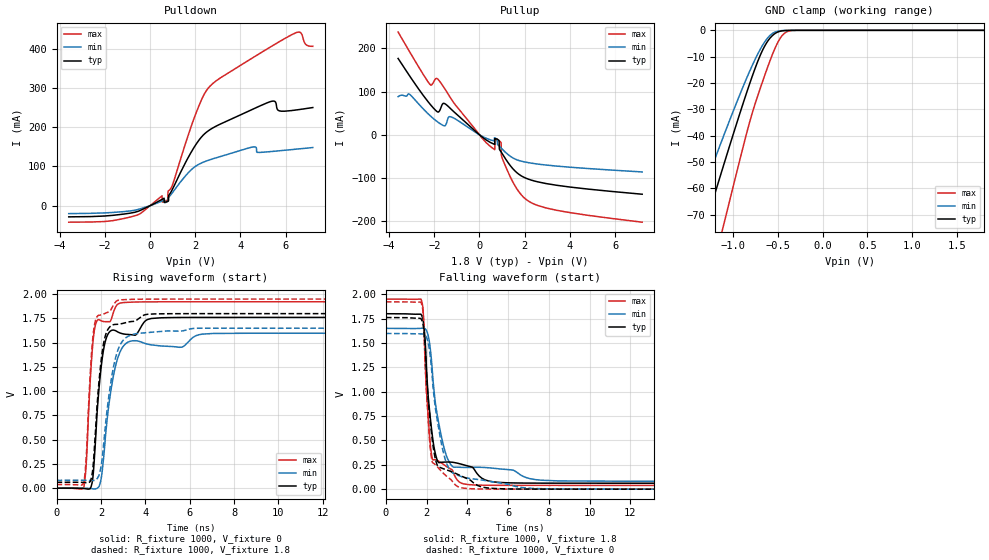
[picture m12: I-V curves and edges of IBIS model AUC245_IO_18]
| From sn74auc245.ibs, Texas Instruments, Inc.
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[Model]   AUC245_IO_18
Model_type  3-state
Enable   Active-Low
Vref =   0
Rref =   1000
Cref =   30p
Vmeas =   0.9
| variable   typ   min   max
C_comp   6.62pF   5.91pF   6.95pF
| C_pullup   7.05pF   0.21pF   13.03pF
| C_pulldown   7.18pF   2.24pF   14.68pF
| C_tri-state   6.62pF   5.91pF   6.95pF
[Temperature Range]   40   100   -40
| Ambient temperature   25   85   -40
[Voltage range]   1.8   1.65   1.95
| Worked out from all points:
|   slope of the pulldown table from 0 to 0.27 V, typ, clamps not added: 34.2 ohm
|   slope of the pullup table from 0 to 0.27 V, typ, clamps not added: 24.6 ohm
|   GND clamp passes 1 mA (typ) near -0.52 V on its own axis
|   rising waveform, R_fixture 1000, V_fixture 0: 20-80 % time 388ps typ, 555ps min, 285ps max; typ from 0 V to 1.76 V
|   falling waveform, R_fixture 1000, V_fixture 1.8: 20-80 % time 438ps typ, 661ps min, 314ps max; typ from 1.8 V to 0.061 V
|   rising waveform, R_fixture 1000, V_fixture 1.8: 20-80 % time 385ps typ, 555ps min, 280ps max; typ from 0.061 V to 1.8 V
|   falling waveform, R_fixture 1000, V_fixture 0: 20-80 % time 445ps typ, 672ps min, 313ps max; typ from 1.76 V to 0 V
[GND Clamp]
| AUC245_IO_18
|   Voltage   I(typ)   I(min)   I(max)
-3.6V     -336.3mA   -280.4mA   -411.7mA
-1.475V   -92.51mA   -73.75mA   -124.5mA
-1.34V    -77.23mA   -61.22mA   -106mA
-1.295V   -72.17mA   -57.08mA   -99.79mA
-1.1V     -50.45mA   -39.48mA   -72.99mA
-830mV    -21.69mA   -16.64mA   -36.59mA
-680mV    -8.152mA   -6.159mA   -20.29mA
-600mV    -3.457mA   -2.337mA   -12.58mA
-520mV    -951.5uA   -506.2uA   -5.863mA
-420mV    -86.5uA    -50.43uA   -943.1uA
-300mV    -2.47uA    -3.001uA   -18.45uA
1.8V      714.1pA    50.2nA     788.2pA
[Pulldown]
| AUC245_IO_18
|   Voltage   I(typ)   I(min)   I(max)
-3.6V     -28.49mA   -20.22mA   -42.08mA
-1.155V   -21.32mA   -15.05mA   -32.66mA
530mV     16.28mA    11.83mA    25.26mA
780mV     11.04mA    10.74mA    14.1mA
800mV     11.66mA    11.63mA    36.72mA
1.97V     150.9mA    98.78mA    226.4mA
2.645V    193.6mA    117.1mA    304.4mA
4.56V     246.4mA    149.8mA    377.8mA
5.38V     266.3mA    138.2mA    406.7mA
5.71V     242mA      140mA      417.9mA
6.445V    244mA      144mA      440.9mA
7.2V      250.3mA    148.3mA    406.4mA
[Pullup]
| AUC245_IO_18
|   Voltage   I(typ)   I(min)   I(max)
-3.6V     176.5mA    88.25mA    237.5mA
-2.185V   70.84mA    44.34mA    116.3mA
-1.835V   52.55mA    29.22mA    128.3mA
-1.53V    71.89mA    20.76mA    106.1mA
-1.26V    59.61mA    41.57mA    83.77mA
480mV     -17.54mA   -11.58mA   -26.82mA
845mV     -12.04mA   -24.63mA   -13.29mA
940mV     -38.16mA   -29.53mA   -16.81mA
980mV     -41.36mA   -31.67mA   -49.57mA
1.26V     -63.84mA   -45.45mA   -85.39mA
2.065V    -100.5mA   -63.4mA    -149.4mA
7.2V      -137.3mA   -85.82mA   -202mA
[Ramp]
| AUC245_IO_18
| variable   typ   min   max
dV/dt_r   1.06/3.92E-10   0.96/5.60E-10   1.16/2.93E-10
dV/dt_f   1.04/4.43E-10   0.94/6.67E-10   1.15/3.23E-10
R_load = 1000
[Rising Waveform]
| AUC245_IO_18
R_fixture =   1000
C_fixture =   0
L_fixture =   0
V_fixture =   0
V_fixture_min = 0
V_fixture_max = 0
|   Time   V(typ)   V(min)   V(max)
0s        11.26nV    38.5nV     1.726nV
1.235ns   -3.215mV   815.2uV    15.23mV
1.335ns   -6.28mV    825.8nV    235.8mV
1.625ns   82.37mV    -5.697mV   1.463V
1.92ns    1.041V     19.16mV    1.737V
2.26ns    1.559V     662.8mV    1.717V
2.55ns    1.63V      1.141V     1.803V
2.86ns    1.6V       1.404V     1.908V
7.04ns    1.761V     1.595V     1.922V
34.99ns   1.761V     1.597V     1.922V
[Falling Waveform]
| AUC245_IO_18
R_fixture =   1000
C_fixture =   0
L_fixture =   0
V_fixture =   1.8
V_fixture_min = 1.65
V_fixture_max = 1.95
|   Time   V(typ)   V(min)   V(max)
0s        1.8V       1.65V      1.95V
1.725ns   1.793V     1.65V      1.948V
1.83ns    1.729V     1.651V     1.824V
2.065ns   985.1mV    1.584V     785.7mV
2.28ns    548.4mV    1.211V     309.5mV
2.545ns   285.7mV    734mV      292mV
2.945ns   278.3mV    358.7mV    236.6mV
3.805ns   250.2mV    223mV      54.87mV
6ns       65.19mV    200.6mV    39.11mV
34.99ns   61.1mV     81.05mV    38.7mV
[Rising Waveform]
| AUC245_IO_18
R_fixture =   1000
C_fixture =   0
L_fixture =   0
V_fixture =   1.8
V_fixture_min = 1.65
V_fixture_max = 1.95
|   Time   V(typ)   V(min)   V(max)
0s        61.05mV    81.01mV    38.68mV
1.235ns   59.16mV    81.79mV    61.05mV
1.335ns   57.48mV    81.3mV     302.7mV
1.62ns    167.6mV    79.35mV    1.513V
1.905ns   1.074V     128.5mV    1.783V
2.225ns   1.589V     696.4mV    1.806V
2.52ns    1.683V     1.192V     1.869V
2.805ns   1.691V     1.447V     1.939V
6.38ns    1.8V       1.649V     1.95V
34.99ns   1.8V       1.65V      1.95V
[Falling Waveform]
| AUC245_IO_18
R_fixture =   1000
C_fixture =   0
L_fixture =   0
V_fixture =   0
V_fixture_min = 0
V_fixture_max = 0
|   Time   V(typ)   V(min)   V(max)
0s        1.761V     1.597V     1.922V
1.725ns   1.748V     1.593V     1.916V
1.82ns    1.693V     1.591V     1.821V
1.89ns    1.568V     1.586V     1.503V
2.11ns    837mV      1.465V     601mV
2.265ns   524.3mV    1.174V     285.4mV
2.515ns   248.9mV    716.2mV    231.7mV
2.88ns    204.9mV    328.8mV    151.6mV
3.67ns    138mV      131.4mV    15.9mV
34.99ns   51.58uV    42.55uV    15.24uV
